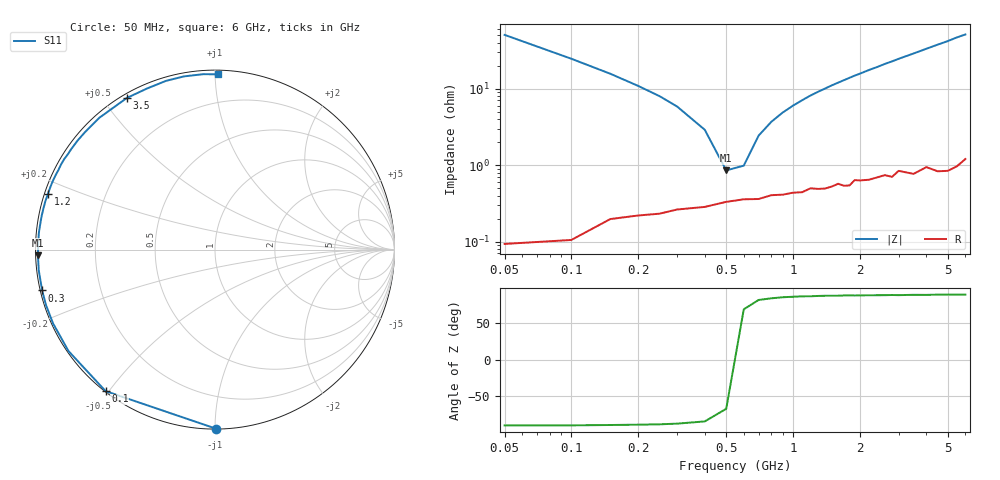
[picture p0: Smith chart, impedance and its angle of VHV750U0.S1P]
! Infineon Technologies  Discrete & RF Semiconductors
! BB 814
! Si Tuning Diode in SOT23
! VR = 0.75 V
! S-Parameters:  July  1999
# GHz  S  MA  R  50
!  f  S11
! GHz  MAG  ANG
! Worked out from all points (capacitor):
!   34 points, 50 MHz to 6 GHz, reference 50 ohm
!   read as one part to ground: C = 62.7 pF near 50 MHz
!   lowest |Z| = 852 mohm at 500 MHz (marker M1)
!   series resonance near 546.2 MHz, so ESL is about 1.4 nH
!   S11 on the Smith chart (normalised r, x): 50 MHz: 0.00, -1.01; 100 MHz: 0.00, -0.49; 300 MHz: 0.01, -0.12; 1.2 GHz: 0.01, +0.16; 3.5 GHz: 0.02, +0.57; 6 GHz: 0.02, +1.02
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0.05  0.9981 -89.6
0.1  0.9966 -127.7
0.15  0.9928 -145.3
0.2  0.9917 -155.5
0.25  0.991 -161.9
0.3  0.9897 -166.7
0.4  0.9887 -173.4
0.5  0.9869 -178.2
0.6  0.9858 177.9
0.7  0.9857 174.5
0.8  0.984 171.6
1  0.983 166.4
1.2  0.9808 161.6
1.4  0.9811 157.3
1.6  0.9787 153.1
1.8  0.98 149.1
1.9  0.9768 147.1
2.2  0.9773 141.5
2.4  0.9762 138.1
2.6  0.9752 134.4
2.8  0.977 131.2
3  0.9732 127.8
3.5  0.9772 120.2
4  0.9742 112.9
4.5  0.979 106.2
5  0.9804 100.2
5.5  0.9796 93.9
6  0.9767 88.9
